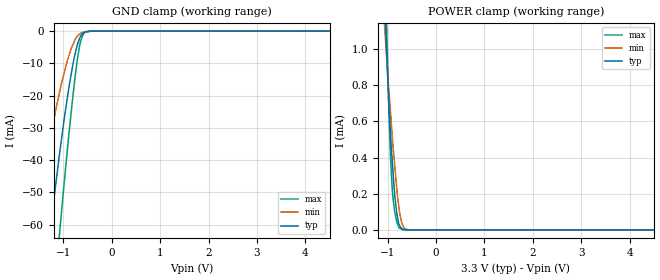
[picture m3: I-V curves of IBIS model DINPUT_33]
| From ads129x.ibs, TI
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|   DINPUT 3.3V Model
[Model]   DINPUT_33
Model_type   Input
|for all products
|Signals   DIN, CLKSEL, START, _CS, _RESET, _PWDN, RESV1
Vinl = 0.66
Vinh = 2.64
|   typ   min   max
|   (nom PVT)   (Fast PVT)   (slow PVT)
|C_comp from frequency sweep method (F=64MHz)
|C_comp   2.2874600e-12   1.7279600e-12   2.8419150e-12
|C_comp from LC tank measurement(L=1nH)
C_comp   1.652E-12   1.343E-12   1.968E-12
| Where   nom PVT is  Nominal Process, 3.3V, 27C
|   Fast PVT is Strong Process, 3.6V, -40C
|   Slow PVT is Weak Process, 3V, 85C
[Voltage Range]   3.3   3   3.6
[Temperature Range]   27   85   -40
[Power Clamp Reference]   3.3   3   3.6
[GND Clamp Reference]   0   0   0
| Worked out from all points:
|   GND clamp passes 1 mA (typ) near -0.62 V on its own axis
|   POWER clamp passes 1 mA (typ) near -1.02 V on its own axis
[GND Clamp]
|   Voltage   I(typ)   I(min)   I(max)
-3.3V     -365.5mA   -258.9mA   -460.2mA
-1.597V   -106mA     -62.12mA   -153.3mA
-1.296V   -64.68mA   -35.02mA   -99.72mA
-1.202V   -52.57mA   -27.66mA   -83.32mA
-1.089V   -38.89mA   -19.5mA    -64.05mA
-1.054V   -34.94mA   -17.04mA   -58.12mA
-812mV    -10.83mA   -4.451mA   -21.03mA
-706.7mV  -3.936mA   -1.508mA   -8.155mA
-630.7mV  -1.241mA   -525.7uA   -2.473mA
-554.3mV  -267.8uA   -311.7uA   -396.5uA
-426.7mV  -11.62uA   -13.55uA   -7.153uA
6.59V     0A         0A         0A
[POWER Clamp]
|   Voltage   I(typ)   I(min)   I(max)
-3.3V     30.92mA    25.65mA    38.05mA
-1.057V   1.262mA    1.102mA    1.572mA
-1.022V   988.4uA    952.9uA    1.141mA
-1.015V   943.9uA    924uA      1.063mA
-972.9mV  681.5uA    762.7uA    640.3uA
-942.5mV  532.8uA    652.4uA    408.8uA
-901.3mV  364.2uA    503.2uA    211.4uA
-859.7mV  209.7uA    372.2uA    108.6uA
-812mV    91.53uA    228.1uA    43.91uA
-750.2mV  23.25uA    90.32uA    9.292uA
-689.4mV  5.727uA    26.05uA    923.4nA
6.59V     0A         0A         0A
